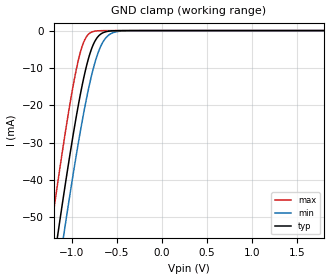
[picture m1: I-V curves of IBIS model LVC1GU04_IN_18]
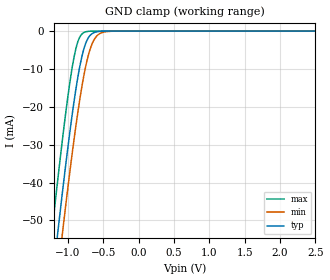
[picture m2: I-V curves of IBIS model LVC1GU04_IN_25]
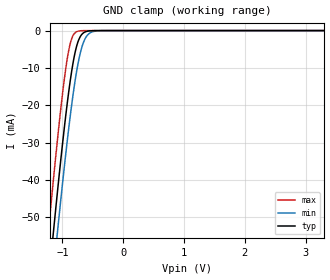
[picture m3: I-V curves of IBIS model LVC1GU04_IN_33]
| TEXAS INSTRUMENTS INCORPORATED
| Standard Linear and Logic Group
| IBIS Model of SN74LVC1GU04
| SINGLE INVERTER GATE
| This file contains package information for the following:
|  SOT 5-pin (DCK) package as [Component] LVC1GU04_DCK
|  SOT 5-pin (DBV) package as [Component] LVC1GU04_DBV
|  SON 6-pin (DRY) package as [Component] LVC1GU04_DRY
|  SON 6-pin (DSF) package as [Component] LVC1GU04_DSF
|  NanoFree WCSP 5-pin (YZP) package as [Component] LVC1GU04_YZP
|  DSBGA 4-pin (YZV) package as [Component] LVC1GU04_YZV
| This device can be powered at the following Vccs:
|  1.8 volt Vcc
|  2.5 volt Vcc
|  3.3 volt Vcc
|  5 volt Vcc
| This file provides unique models under the [Model Selector] for each Vcc.
| For operation at a specific Vcc, select the appropriate model after each
| [Model Selector] keyword.
[IBIS Ver]   3.2
[Comment char]  |_char
[File Name]   sn74lvc1gu04.ibs
[File Rev]   1.2 | a_die
[Date]   December 22, 2005
[Source]   Data created from TI-SPICE simulations at TI-SLL.
[Notes]   The following is an IBIS list for the SN74LVC1GU04.
   Please contact sllibis@ti.com with questions and
   comments concerning SLL IBIS models.
   - FILE REV HISTORY
   - 1.2 YEP, YZP, and YZV packages added on 12/22/05
   - C_comp values are taken at a different test condition than
   the Ci in data sheet.
   - Power clamp data deleted as there is no power-clamp diode.
[Disclaimer] Property of Texas Instruments Incorporated. Unauthorized
   reproduction and/or distribution is strictly prohibited.
   This product is protected under copyright law.
   Created 2002,(C) Copyright 2002, Texas Instruments
   Incorporated, All Rights Reserved
   UNLESS THERE IS A SIGNED, WRITTEN AGREEMENT TO THE
   CONTRARY, TEXAS INSTRUMENTS (TI) IS PROVIDING THE IBIS
   MODELS  AND WITHOUT ANY WARRANTY, EXPRESSED OR
   IMPLIED. TI assumes no liability for:
   1) the accuracy of the IBIS models provided to your
   company;
   2) the proper functioning of these IBIS Models in your
   design or for any resulting applications; or
   3) infringement of patents, copyrights or intellectual
   property rights resulting from your use of these IBIS
   models.
   TI provides IBIS Models as a service to our customers.
   You and your company shall not distribute, sell or give
   these models to anyone else without prior written
   permission from TI.
   TI reserves the right to make changes to our products or
   to discontinue any semiconductor product or service
   without notice, and advises our customers to obtain the
   latest version of relevant information to verify, before
   placing orders, that the information being relied on is
   current.
   Please be aware that your receipt and use of the IBIS
   information provided shall serve as acceptance of these
   terms and conditions. If you do not accept these terms,
   you should return or destroy the IBIS models and any
   other accompanying information immediately.
| Component LVC1GU04_DCK 5-pin SOT
[Component]   LVC1GU04_DCK
[Manufacturer]   Texas Instruments, Inc.
[Package]
|   typ   min   max
R_pkg   2.000e-02   1.700e-02   2.500e-02
L_pkg   9.980e-10   8.810e-10   1.069e-09
C_pkg   1.460e-13   1.180e-13   2.050e-13
[Pin]   signal_name   model_name   R_pin   L_pin   C_pin
1   NC   NC   1.900e-02   1.069e-09   1.620e-13
2   A   LVC1GU04_IN   1.800e-02   8.810e-10   1.210e-13
3   GND   GND   1.700e-02   1.031e-09   2.050e-13
4   Y   LVC1GU04_OUT   2.000e-02   9.600e-10   1.240e-13
5   VCC   POWER   2.500e-02   1.049e-09   1.180e-13
| Component LVC1GU04_DBV 5-pin SOT
[Component]   LVC1GU04_DBV
[Manufacturer]   Texas Instruments, Inc.
[Package]
|   typ   min   max
R_pkg   2.500e-02   2.100e-02   2.900e-02
L_pkg   1.529e-09   1.312e-09   1.906e-09
C_pkg   1.560e-13   1.100e-13   2.400e-13
[Pin]   signal_name   model_name   R_pin   L_pin   C_pin
1   NC   NC   2.100e-02   1.511e-09   1.440e-13
2   A   LVC1GU04_IN   2.300e-02   1.312e-09   1.380e-13
3   GND   GND   2.900e-02   1.906e-09   2.400e-13
4   Y   LVC1GU04_OUT   2.600e-02   1.541e-09   1.500e-13
5   VCC   POWER   2.500e-02   1.374e-09   1.100e-13
| Component LVC1GU04_DSF 6-pin SON
[Component]   LVC1GU04_DSF
[Manufacturer]   Texas Instruments, Inc.
[Package]
|   typ   min   max
R_pkg   2.42E-02   1.03E-03   4.06E-02
L_pkg   2.78E-10   1.77E-11   4.71E-10
C_pkg   1.00E-13   7.41E-14   1.18E-13
[Pin]   signal_name   model_name   R_pin   L_pin   C_pin
1   NC   NC   3.06E-03   1.77E-11   7.41E-14
2   A   LVC1GU04_IN   2.78E-02   3.07E-10   1.06E-13
3   GND   GND   3.67E-02   4.23E-10   1.14E-13
4   Y   LVC1GU04_OUT   4.06E-02   4.71E-10   1.18E-13
5   NC   NC   1.03E-03   3.45E-11   7.65E-14
6   VCC   POWER   3.63E-02   4.13E-10   1.13E-13
| Component LVC1GU04_DRY 5-pin NanoFree WCSP
[Component]   LVC1GU04_DRY
[Manufacturer]   Texas Instruments, Inc.
[Package]
|   typ   min   max
R_pkg   2.82E-02   1.03E-03   4.61E-02
L_pkg   3.23E-10   1.45E-11   5.34E-10
C_pkg   1.04E-13   7.41E-14   1.22E-13
[Pin]   signal_name   model_name   R_pin   L_pin   C_pin
1   NC   NC   1.03E-03   1.46E-11   7.41E-14
2   A   LVC1GU04_IN   3.22E-02   3.49E-10   1.09E-13
3   GND   GND   4.46E-02   5.18E-10   1.21E-13
4   Y   LVC1GU04_OUT   4.61E-02   5.34E-10   1.22E-13
5   NC   NC   1.03E-03   1.45E-11   7.65E-14
6   VCC   POWER   4.41E-02   5.05E-10   1.20E-13
| Component LVC1GU04_YZP 5-pin NanoFree WCSP
[Component]   LVC1GU04_YZP
[Manufacturer]   Texas Instruments, Inc.
[Package]
|   typ   min   max
R_pkg   0.001   0.001   0.001
L_pkg   0.021nH   0.021nH   0.021nH
C_pkg   0.046pF   0.045pF   0.047pF
[Pin]   signal_name   model_name   R_pin   L_pin   C_pin
1   DNU   NC   0.001   0.021nH   0.046pF
2   A   LVC1GU04_IN   0.001   0.021nH   0.047pF
3   GND   GND   0.001   0.021nH   0.046pF
4   Y   LVC1GU04_OUT   0.001   0.021nH   0.045pF
5   VCC   POWER   0.001   0.021nH   0.045pF
| Component LVC1GU04_YZV 4-pin DSBGA
[Component]   LVC1GU04_YZV
[Manufacturer]   Texas Instruments, Inc.
[Package]
|   typ   min   max
R_pkg   1.000e-03   1.000e-03   1.000e-03
L_pkg   2.600e-11   2.600e-11   2.600e-11
C_pkg   1.400e-14   1.400e-14   1.400e-14
[Pin]   signal_name   model_name   R_pin   L_pin   C_pin
1   A   LVC1GU04_IN   1.000e-03   2.600e-11   1.400e-14
2   GND   GND   1.000e-03   2.600e-11   1.400e-14
3   Y   LVC1GU04_OUT   1.000e-03   2.600e-11   1.400e-14
4   VCC   POWER   1.000e-03   2.600e-11   1.400e-14
| Model LVC1GU04_IN
[Model Selector]   LVC1GU04_IN
LVC1GU04_IN_18   1.8 volt Vcc
LVC1GU04_IN_25   2.5 volt Vcc
LVC1GU04_IN_33   3.3 volt Vcc
LVC1GU04_IN_50   5 volt Vcc
| Model LVC1GU04_OUT
[Model Selector]   LVC1GU04_OUT
LVC1GU04_OUT_18   1.8 volt Vcc
LVC1GU04_OUT_25   2.5 volt Vcc
LVC1GU04_OUT_33   3.3 volt Vcc
LVC1GU04_OUT_50   5 volt Vcc
| Models and submodels in the file (8): LVC1GU04_IN_18 (Input), LVC1GU04_IN_25 (Input), LVC1GU04_IN_33 (Input), LVC1GU04_IN_50 (Input), LVC1GU04_OUT_18 (Output), LVC1GU04_OUT_25 (Output), LVC1GU04_OUT_33 (Output), LVC1GU04_OUT_50 (Output)
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[Model]   LVC1GU04_IN_18
Model_type  Input
Vinl=0.4125
Vinh=1.4625
| variable   typ   min   max
C_comp   3.64pF   1.74pF   4.47pF
[Temperature Range]   40   100   -40
| Ambient temperature   25   85   -40
[Voltage range]   1.8   1.65   1.95
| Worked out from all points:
|   GND clamp passes 1 mA (typ) near -0.68 V on its own axis
[GND Clamp]
| LVC1GU04_IN_18
|   Voltage   I(typ)   I(min)   I(max)
-5.5V     -872.3mA   -880mA     -863mA
-1.235V   -68.47mA   -79.32mA   -54.53mA
-1.155V   -55.02mA   -65.9mA    -41.02mA
-1.09V    -44.44mA   -55.28mA   -30.51mA
-1.07V    -41.27mA   -52.08mA   -27.39mA
-955mV    -24.08mA   -34.45mA   -11.33mA
-865mV    -12.71mA   -22.05mA   -3.093mA
-745mV    -3.048mA   -8.978mA   -175.9uA
-670mV    -836.3uA   -3.901mA   -23.18uA
-590mV    -176.2uA   -1.257mA   -2.616uA
-340mV    -1.112uA   -19.62uA   -2.839nA
1.8V      1.111nA    59.61nA    3.29pA
[Model]   LVC1GU04_IN_25
Model_type  Input
Vinl=0.575
Vinh=2.025
| variable   typ   min   max
C_comp   4.02pF   2.56pF   4.84pF
[Temperature Range]   40   100   -40
| Ambient temperature   25   85   -40
[Voltage range]   2.5   2.3   2.7
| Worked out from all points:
|   GND clamp passes 1 mA (typ) near -0.68 V on its own axis
[GND Clamp]
| LVC1GU04_IN_25
|   Voltage   I(typ)   I(min)   I(max)
-5.5V     -872.3mA   -880mA     -863mA
-1.23V    -67.62mA   -78.47mA   -53.67mA
-1.155V   -55.02mA   -65.9mA    -41.02mA
-1.13V    -50.91mA   -61.78mA   -36.92mA
-1.085V   -43.65mA   -54.48mA   -29.72mA
-1.065V   -40.48mA   -51.28mA   -26.62mA
-950mV    -23.39mA   -33.72mA   -10.74mA
-860mV    -12.16mA   -21.41mA   -2.808mA
-785mV    -5.383mA   -12.75mA   -501uA
-715mV    -1.873mA   -6.62mA    -78.61uA
-575mV    -130.5uA   -995.5uA   -1.737uA
2.5V      1.112nA    59.61nA    4.652pA
[Model]   LVC1GU04_IN_33
Model_type  Input
Vinl=0.75
Vinh=2.7
| variable   typ   min   max
C_comp   4.19pF   2.71pF   4.91pF
[Temperature Range]   40   100   -40
| Ambient temperature   25   85   -40
[Voltage range]   3.3   3   3.6
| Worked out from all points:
|   GND clamp passes 1 mA (typ) near -0.68 V on its own axis
[GND Clamp]
| LVC1GU04_IN_33
|   Voltage   I(typ)   I(min)   I(max)
-5.5V     -872.3mA   -880mA     -863mA
-1.235V   -68.47mA   -79.32mA   -54.53mA
-1.155V   -55.02mA   -65.9mA    -41.02mA
-1.13V    -50.91mA   -61.78mA   -36.92mA
-1.085V   -43.65mA   -54.48mA   -29.72mA
-960mV    -24.78mA   -35.18mA   -11.94mA
-865mV    -12.71mA   -22.05mA   -3.093mA
-790mV    -5.74mA    -13.27mA   -568.9uA
-715mV    -1.873mA   -6.62mA    -78.61uA
-645mV    -520uA     -2.804mA   -11.73uA
-565mV    -106.8uA   -850.2uA   -1.322uA
3.3V      1.114nA    59.61nA    6.193pA
